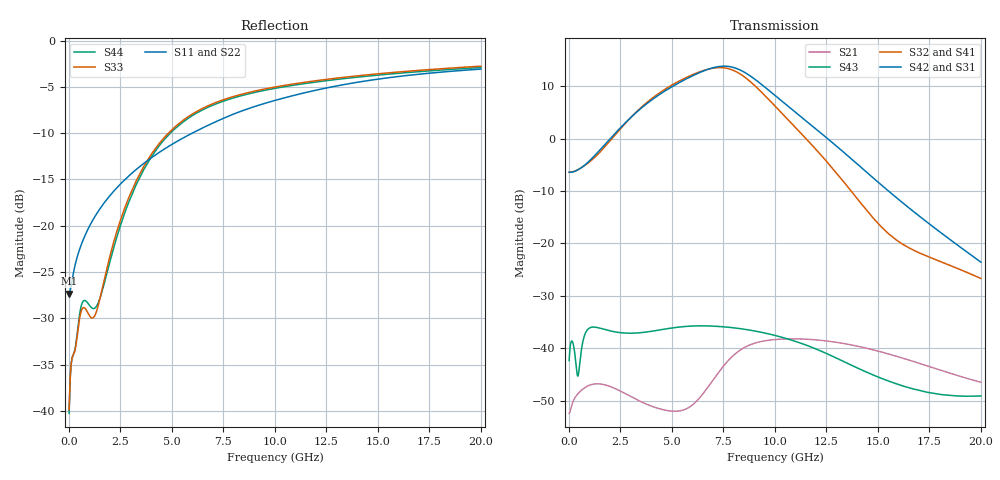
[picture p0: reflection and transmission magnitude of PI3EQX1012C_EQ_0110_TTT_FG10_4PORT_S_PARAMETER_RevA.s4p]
! NPort=4 DATA=2000 NOISE=0 GROUPDELAY=0 COMPLEX_DATAFORMAT=POLAR
! NumOfBlock=1 NumOfParam=0
! .MODEL Smodel S TSTONEFILE=PI3EQX1012C_EQ_0110_TTT_FG10_4PORT_S_PARAMETER_RevA.s4p TYPE=S
!  -- The above .MODEL line can be used for the S element in the netlist.
! The s parameter is extracted from the linear redriver, it is not bi-directional; only s(4,1)s(4,2) and s(3,1)s(3,2)
! should be the insertion loss
!Port definition:
!Port1 = input+
!Port2 = input-
!Port3 = output+
!Port4 = output-
# Hz S MA R  50
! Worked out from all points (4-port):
!   2000 points, 10 MHz to 20 GHz, reference 50 ohm
!   strongest paths, dB at 10 MHz, 5.01 GHz, 10.01 GHz, 15.01 GHz, 20 GHz:
!     S42: -6.4, 9.9, 8.2, -8.3, -23.6
!     S31: -6.4, 9.9, 8.2, -8.5, -24.0
!     S32: -6.4, 10.3, 6.2, -16.2, -26.7
!     S41: -6.4, 10.3, 6.4, -16.4, -27.0
!     S43: -42.4, -36.1, -37.6, -45.5, -49.1
!     S21: -52.4, -52.0, -38.4, -40.6, -46.5
!   lowest |S11| = -27.3 dB at 10 MHz (marker M1), VSWR 1.09, Z = 45.9 - j0.123 ohm
!   |S11| at or under -10 dB: start of sweep to 5.986 GHz
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1e7  0.04301 -178.2  0.002379 1.5  0.0008102 -0.5  0.0008039 -0.5
     0.002388 1.5  0.04109 -178.1  0.000927 -0.5  0.0009197 -0.5
     0.4784 -0.1  0.4775 180.0  0.01016 -4.0  0.007598 -25.7
     0.4771 179.9  0.4794 -0.2  0.007615 -25.8  0.009722 -4.0
4.11e9  0.2373 -124.3  0.002781 0.1  0.0003806 -56.9  0.0003788 -57.2
        0.00275 0.3  0.241 -123.2  0.0004326 -57.5  0.0004306 -57.9
        2.416 -63.2  2.491 127.4  0.2534 -83.7  0.01361 33.6
        2.478 128.1  2.413 -61.6  0.0146 30.6  0.2455 -83.4
5.75e9  0.3065 -123.8  0.002724 37.5  0.0002775 -58.3  0.0002764 -59.3
        0.002666 36.0  0.3115 -123.1  0.0003147 -59.3  0.0003134 -60.2
        3.75 -130.0  3.88 60.3  0.3854 -99.5  0.01639 9.4
        3.895 60.6  3.765 -128.0  0.01616 6.8  0.3776 -99.2
7.05e9  0.3611 -124.4  0.005374 57.7  0.0002395 -55.9  0.0002375 -57.2
        0.005137 58.1  0.3666 -123.9  0.0002702 -57.1  0.000268 -58.4
        4.757 166.6  4.729 -3.7  0.459 -109.5  0.0167 -10.8
        4.77 -3.8  4.785 168.7  0.01622 -11.9  0.4508 -109.4
8.18e9  0.4084 -125.8  0.009433 42.2  0.0002238 -54.2  0.0002207 -55.7
        0.00917 43.5  0.4143 -125.4  0.0002508 -55.5  0.0002474 -57.0
        4.616 102.3  4.299 -67.9  0.5057 -116.3  0.01584 -26.2
        4.352 -68.4  4.646 104.6  0.01549 -26.7  0.4971 -116.1
9.53e9  0.4587 -128.1  0.01193 14.9  0.000214 -53.9  0.0002099 -55.4
        0.01177 16.2  0.4656 -127.6  0.0002381 -55.0  0.0002337 -56.6
        3.065 33.4  2.561 -135.3  0.5482 -122.4  0.01421 -42.3
        2.601 -136.3  3.087 36.1  0.01392 -42.9  0.5395 -122.3
2e10  0.7013 -144.6  0.004785 -70.3  0.0001465 -72.3  0.0001414 -73.8
      0.004726 -69.5  0.7163 -144.4  0.0001624 -72.1  0.0001567 -73.8
      0.06306 105.9  0.04628 32.6  0.7272 -143.5  0.003578 -51.6
      0.04456 30.8  0.0663 110.7  0.003497 -48.9  0.7152 -143.3
